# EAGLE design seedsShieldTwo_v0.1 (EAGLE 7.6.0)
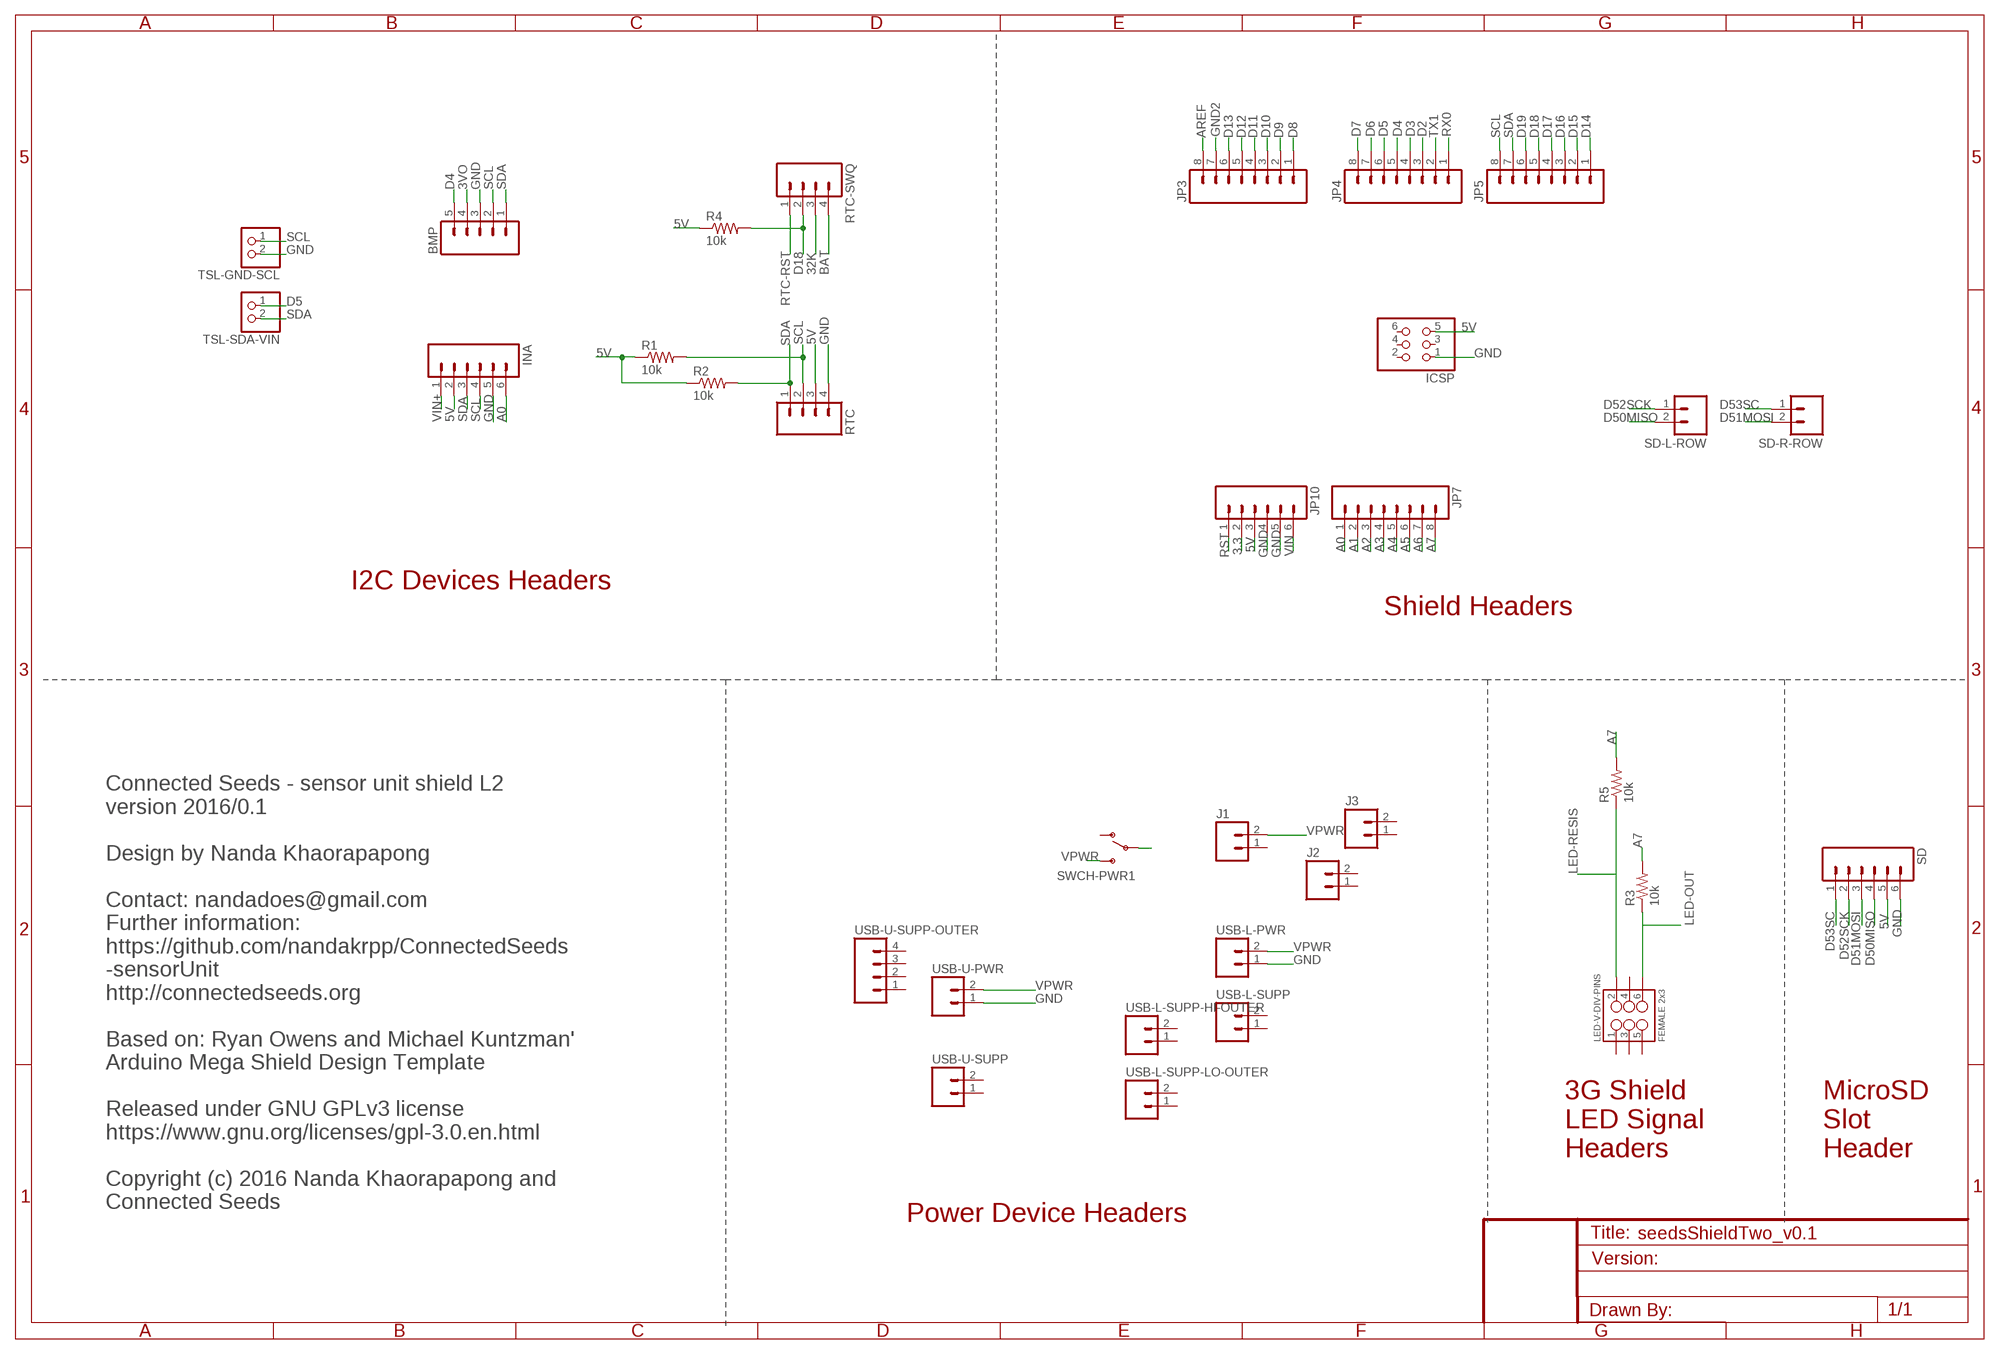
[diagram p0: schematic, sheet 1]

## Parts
BMP  M05PTH  [1X05]
ICSP  PINHD-2X3  [2X03]
INA  M06LOCK  [1X06_LOCK]
J1  M02LOCK_LONGPADS  [1X02_LOCK_LONGPADS]
J2  M02LOCK_LONGPADS  [1X02_LOCK_LONGPADS]
J3  M02LOCK_LONGPADS  [1X02_LOCK_LONGPADS]
JP3  M08LOCK  [1X08_LOCK]
JP4  M08LOCK  [1X08_LOCK]
JP5  M08LOCK  [1X08_LOCK]
JP7  M08LOCK  [1X08_LOCK]
JP10  M06LOCK  [1X06_LOCK]
LED-V-DIV-PINS  FEMALE 2x3  M03X2FEMALE  [2X3]
R1  10k  RESISTORPTH-1/4W  [AXIAL-0.4]
R2  10k  RESISTORPTH-1/4W  [AXIAL-0.4]
R3  10k  RESISTORPTH-1/4W  [AXIAL-0.4]
R4  10k  RESISTORPTH-1/4W  [AXIAL-0.4]
R5  10k  RESISTORPTH-1/4W  [AXIAL-0.4]
RTC  M04PTH  [1X04]
RTC-SWQ  M04PTH  [1X04]
SD  M06LOCK  [1X06_LOCK]
SD-L-ROW  M02PTH  [1X02]
SD-R-ROW  M02PTH  [1X02]
SWCH-PWR1  SWITCH-SPDTPTH_LOCK  [SWITCH-SPDT_LOCK.007S]
TSL-GND-SCL  JST_2PIN-THM  [JST-PH-2-THM]
TSL-SDA-VIN  JST_2PIN-THM  [JST-PH-2-THM]
USB-L-PWR  M02PTH  [1X02]
USB-L-SUPP  M02PTH  [1X02]
USB-L-SUPP-HI-OUTER  M02PTH  [1X02]
USB-L-SUPP-LO-OUTER  M02PTH  [1X02]
USB-U-PWR  M02PTH  [1X02]
USB-U-SUPP  M02PTH  [1X02]
USB-U-SUPP-OUTER  M04LOCK  [1X04_LOCK]

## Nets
3.3: JP10.2
3VO: BMP.4
5V: ICSP.5 INA.2 JP10.3 R1.P$1 R2.P$1 R4.P$1 RTC.3 SD.5
32K: RTC-SWQ.3
A0: INA.6 JP7.1
A1: JP7.2
A2: JP7.3
A3: JP7.4
A4: JP7.5
A5: JP7.6
A6: JP7.7
A7: JP7.8 R3.P$2 R5.P$2
AREF: JP3.8
BAT: RTC-SWQ.4
D2: JP4.3
D3: JP4.4
D4: BMP.5 JP4.5
D5: JP4.6 TSL-SDA-VIN.1
D6: JP4.7
D7: JP4.8
D8: JP3.1
D9: JP3.2
D10: JP3.3
D11: JP3.4
D12: JP3.5
D13: JP3.6
D14: JP5.1
D15: JP5.2
D16: JP5.3
D17: JP5.4
D18: JP5.5 R4.P$2 RTC-SWQ.2
D19: JP5.6
D50MISO: SD-L-ROW.2 SD.4
D51MOSI: SD-R-ROW.2 SD.3
D52SCK: SD-L-ROW.1 SD.2
D53SC: SD-R-ROW.1 SD.1
GND: BMP.3 ICSP.1 INA.5 JP10.4 JP10.5 RTC.4 SD.6 TSL-GND-SCL.2 USB-L-PWR.1 USB-U-PWR.1
GND2: JP3.7
LED-OUT: LED-V-DIV-PINS.6 R3.P$1
LED-RESIS: LED-V-DIV-PINS.2 R5.P$1
RST: JP10.1
RTC-RST: RTC-SWQ.1
RX0: JP4.1
SCL: BMP.2 INA.4 JP5.8 R1.P$2 RTC.2 TSL-GND-SCL.1
SDA: BMP.1 INA.3 JP5.7 R2.P$2 RTC.1 TSL-SDA-VIN.2
TX1: JP4.2
VIN: JP10.6
VIN+: INA.1 SWCH-PWR1.2(P)
VPWR: J1.2 SWCH-PWR1.3(S) USB-L-PWR.2 USB-U-PWR.2
Unconnected: ICSP.2 ICSP.3 ICSP.4 ICSP.6 J1.1 J2.1 J2.2 J3.1 J3.2 LED-V-DIV-PINS.1 LED-V-DIV-PINS.3 LED-V-DIV-PINS.4 LED-V-DIV-PINS.5 SWCH-PWR1.1(O) USB-L-SUPP-HI-OUTER.1 USB-L-SUPP-HI-OUTER.2 USB-L-SUPP-LO-OUTER.1 USB-L-SUPP-LO-OUTER.2 USB-L-SUPP.1 USB-L-SUPP.2 USB-U-SUPP-OUTER.1 USB-U-SUPP-OUTER.2 USB-U-SUPP-OUTER.3 USB-U-SUPP-OUTER.4 USB-U-SUPP.1 USB-U-SUPP.2

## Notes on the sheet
- I2C Devices Headers
- Shield Headers
- 3G Shield
  LED Signal 
  Headers
- MicroSD 
  Slot
  Header
- Connected Seeds - sensor unit shield L2 
  version 2016/0.1                                                                                                        
  
  Design by Nanda Khaorapapong                     
  
  Contact: nandadoes@gmail.com
  Further information:
  https://github.com/nandakrpp/ConnectedSeeds
  -sensorUnit
  http://connectedseeds.org
  
  Based on: Ryan Owens and Michael Kuntzman' 
  Arduino Mega Shield Design Template
  
  Released under GNU GPLv3 license
  https://www.gnu.org/licenses/gpl-3.0.en.html
  
  Copyright (c) 2016 Nanda Khaorapapong and 
  Connected Seeds
- Power Device Headers

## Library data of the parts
BMP = SparkFun-Connectors:M05: Header 5 Standard 5-pin 0.1" header. Use with straight break away headers (SKU : PRT-00116), right angle break away headers (PRT-00553), swiss pins (PRT-00743), machine pins (PRT-00117), and female headers (PRT-00115). Molex polarized connector foot print use with SKU : PRT-08230 with associated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
ICSP = SparkFun-Connectors:PINHD-2X3: PIN HEADER
INA JP10 SD = SparkFun:M06: Header 6 Standard 6-pin 0.1" header. Use with straight break away headers (SKU : PRT-00116), right angle break away headers (PRT-00553), swiss pins (PRT-00743), machine pins (PRT-00117), and female headers (PRT-00115). Molex polarized connector foot print use with SKU : PRT-08094 with associated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
J1-J3 SD-L-ROW SD-R-ROW USB-L-PWR USB-L-SUPP USB-L-SUPP-HI-OUTER USB-L-SUPP-LO-OUTER USB-U-PWR USB-U-SUPP = SparkFun-Connectors:M02: Standard 2-pin 0.1" header. Use with
JP3-JP5 JP7 = SparkFun:M08: Header 8 Standard 8-pin 0.1" header. Use with straight break away headers (SKU : PRT-00116), right angle break away headers (PRT-00553), swiss pins (PRT-00743), machine pins (PRT-00117), and female headers (PRT-00115).
LED-V-DIV-PINS = SparkFun-Connectors:M03X2: 2x3 .1" header. Shrouded, with keying- CONN-10681 SMT- CONN-11415 Pogo pins- HW-11044; PROD_ID: CONN-11566
R1-R5 = SparkFun-Passives:RESISTOR: Resistor
RTC RTC-SWQ USB-U-SUPP-OUTER = SparkFun-Connectors:M04: Header 4 Standard 4-pin 0.1" header. Use with straight break away headers (SKU : PRT-00116), right angle break away headers (PRT-00553), swiss pins (PRT-00743), machine pins (PRT-00117), and female headers (PRT-00115). Molex polarized connector foot print use with SKU : PRT-08231 with associated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; PROD_ID: CONN-09696
SWCH-PWR1 = SparkFun-Electromechanical:SWITCH-SPDT: SPDT Switch Simple slide switch, Spark Fun Electronics SKU : COM-00102 DPDT SMT slide switch, AYZ0202, SWCH-08179
TSL-GND-SCL TSL-SDA-VIN = adafruit:JST_2PIN: JST 2-Pin Connectors of various flavors

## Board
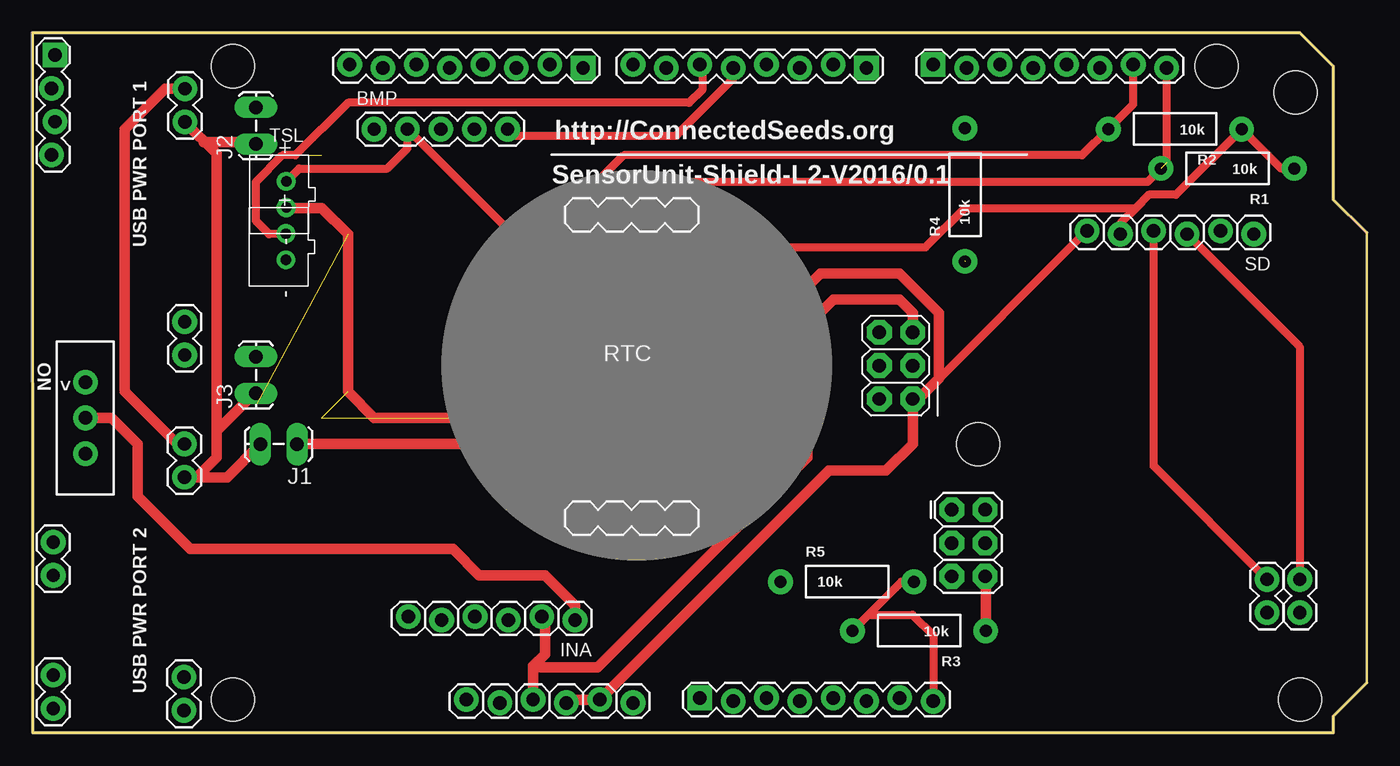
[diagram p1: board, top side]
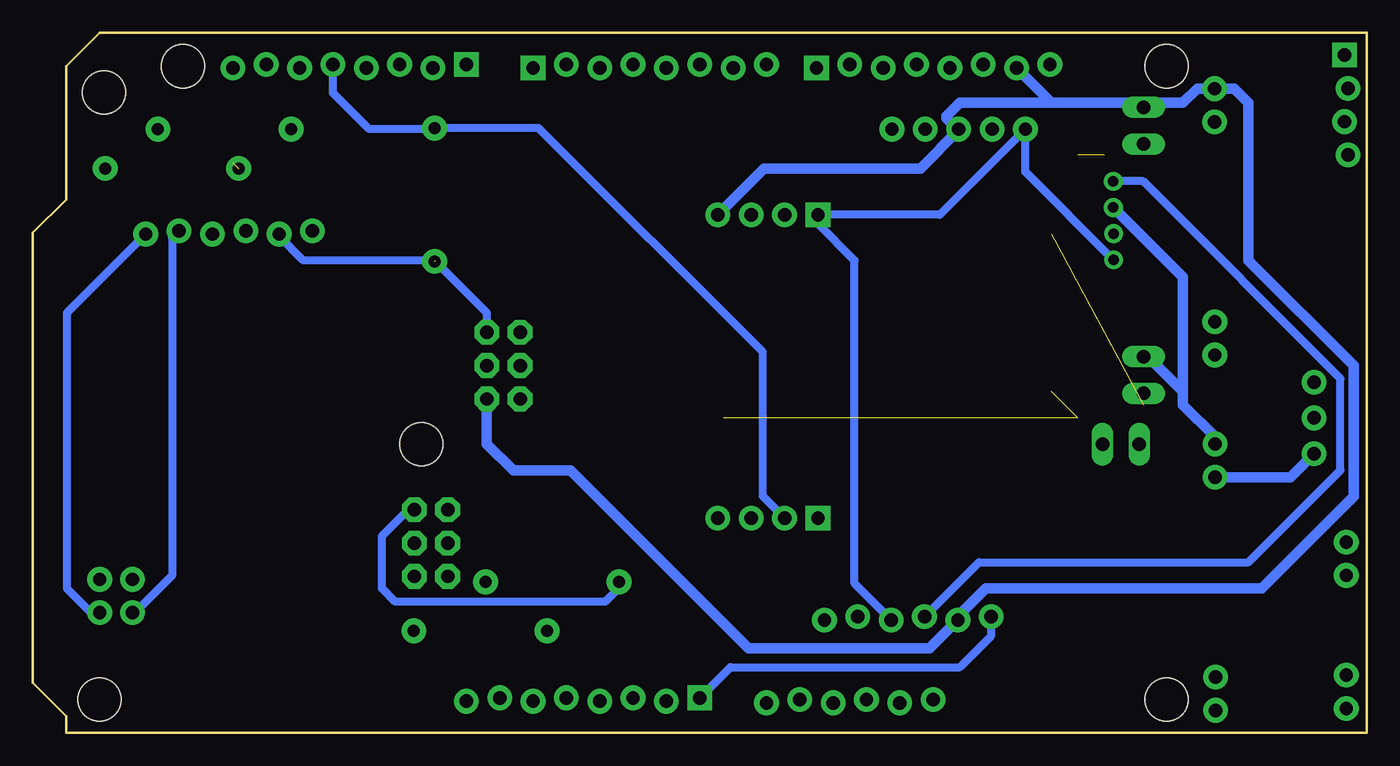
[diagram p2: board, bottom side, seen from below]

Size 101.6 x 53.34 mm. Coordinates in mm from the lower left corner, seen from the top.
Outline: 0,0 99.06,0 99.06,1.27 101.6,3.81 101.6,38.1 99.06,40.64 99.06,50.8 96.52,53.34 0,53.34 0,0
Copper layers (1*16): Top 0.035mm / dielectric 1.5mm / Bottom 0.035mm
Design rules "PCB_TRAIN": minimum track width 8mil, minimum drill 20mil, track to track 8mil, track to pad 8mil, pad to pad 8mil, via to via 8mil, smd to smd 8mil, copper to edge 10mil, drill to drill 8mil, minimum pad ring 12mil, minimum via ring 10mil, stop-mask expansion 4mil, vias tented up to drill 25mil, thermal gap 10mil

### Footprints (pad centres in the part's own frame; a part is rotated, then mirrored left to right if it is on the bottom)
1X05 = drill 1.016 pad 1.88: 1 0,0; 2 2.54,0; 3 5.08,0; 4 7.62,0; 5 10.16,0
2X03 = drill 1.016 pad 1.88 octagon: 1 -2.54,-1.27; 2 -2.54,1.27; 3 0,-1.27; 4 0,1.27; 5 2.54,-1.27; 6 2.54,1.27
1X06_LOCK = drill 1.016 pad 1.88: 1 0,0; 2 2.54,-0.254; 3 5.08,0; 4 7.62,-0.254; 5 10.16,0; 6 12.7,-0.254
1X02_LOCK_LONGPADS = drill 1.016 long: 1 -0.127,0; 2 2.667,0
1X08_LOCK = drill 1.016 pad 1.88 square: 1 0,0.127 | drill 1.016 pad 1.88: 2 2.54,-0.127; 3 5.08,0.127; 4 7.62,-0.127; 5 10.16,0.127; 6 12.7,-0.127; 7 15.24,0.127; 8 17.78,-0.127
2X3 = drill 1.016 pad 1.88 octagon: 1 0,0; 2 0,2.54; 3 2.54,0; 4 2.54,2.54; 5 5.08,0; 6 5.08,2.54
AXIAL-0.4 = drill 0.9 pad 1.88: P$1 -5.08,0; P$2 5.08,0
1X04 = drill 1.016 pad 1.88 square: 1 0,0 | drill 1.016 pad 1.88: 2 2.54,0; 3 5.08,0; 4 7.62,0
1X02 = drill 1.016 pad 1.88: 1 0,0; 2 2.54,0
SWITCH-SPDT_LOCK.007S = drill 1.016 pad 1.88: 1 0,2.718; 2 0,0; 3 0,-2.718
JST-PH-2-THM = drill 0.8 pad 1.422: 1 1,0; 2 -1,0
STAND-OFF = hole 3.302: 0,0
1X04_LOCK = drill 1.016 pad 1.88 square: 1 0,0.127 | drill 1.016 pad 1.88: 2 2.54,-0.127; 3 5.08,0.127; 4 7.62,-0.127

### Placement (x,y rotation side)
BMP  26,46 0 top
ICSP  65.75,27.98 90 top
INA  41.3,8.6 180 top
J1  20,22 180 top
J2  17,45 90 top
J3  17,26 90 top
JP3  41.91,50.8 180 top
JP4  63.5,50.8 180 top
JP5  68.58,50.8 0 top
JP7  50.8,2.54 0 top
JP10  33.02,2.54 0 top
LED-V-DIV-PINS  70,17 270 top
R1  91,43 180 top
R2  87,46 180 top
R3  67.51,7.78 180 top
R4  71,41 90 top
R5  62.03,11.51 0 top
RTC  41.8,39.48 0 top
RTC-SWQ  41.8,16.37 0 top
SD  93,38 180 top
SD-L-ROW  94,9.16 90 top
SD-R-ROW  96.5,9.16 90 top
SWCH-PWR1  4,24 0 top
TSL-GND-SCL  19.3,41.03 90 top
TSL-SDA-VIN  19.28,37.04 90 top
U$1  [STAND-OFF]  15.24,2.54 0 top
U$2  [STAND-OFF]  72,22 90 top
U$3  [STAND-OFF]  15.24,50.8 0 top
U$4  [STAND-OFF]  90.17,50.8 0 top
U$5  [STAND-OFF]  96.17,48.8 0 top
U$6  [STAND-OFF]  96.52,2.54 0 top
USB-L-PWR  11.54,22.01 270 top
USB-L-SUPP  11.52,4.26 270 top
USB-L-SUPP-HI-OUTER  1.55,4.4 270 top
USB-L-SUPP-LO-OUTER  1.55,14.54 270 top
USB-U-PWR  11.58,49.08 270 top
USB-U-SUPP  11.57,31.33 270 top
USB-U-SUPP-OUTER  1.55,51.65 270 top

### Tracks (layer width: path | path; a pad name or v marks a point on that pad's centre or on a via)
5V  (1 unrouted)
  Top 0.61: R1.P$1 95.08,43 R2.P$1 87.08,41 85,41 84,40 | 84,40 82.84,38.84 SD.5 | RTC.3 49.36,37 68,37 71,40 84,40
  Top 0.813: INA.2 39,8.61 39,6 38.1,5.1 38.1,5 | 38.1,5 JP10.3 | 38.1,5 43,5 59,21 59,31 | 21,22 50,22 59,31 | 59,31 61,33 66,33 67.02,31.98 ICSP.5
  Bottom 0.61: SD.5 82.84,37.84 81,36 71,36 67.02,32.02 ICSP.5
A0
  Bottom 0.61: JP7.1 48.47,5 31,5 28.6,7.4 INA.6
A7
  Top 0.61: R5.P$2 66.16,11.51 R3.P$2 63.65,9 67,9 68.58,7.42 JP7.8
D4
  Top 0.61: BMP.5 36.66,45.5 49,45.5 53.34,49.84 JP4.5
D5  (1 unrouted)
  Top 0.61: TSL-SDA-VIN.1 19.25,38 18,38 17,39 17,42 19,44 20,44 24,48 50,48 51,49 51,50.73 JP4.6
D18
  Bottom 0.61: R4.P$2 71.08,46 76,46 78.74,48.74 JP5.5 | 70.08,46.08 R4.P$2 | RTC-SWQ.2 46,18.03 46,29 63.08,46.08 R4.P$2
D50MISO
  Top 0.61: SD-L-ROW.2 85.38,20.32 SD.4
D51MOSI
  Top 0.61: SD.3 96.5,29.42 SD-R-ROW.2
D52SCK
  Bottom 0.61: SD.2 91,37.71 91,12 93.84,9.16 SD-L-ROW.1
D53SC
  Bottom 0.61: SD.1 99,32 99,11 97.16,9.16 SD-R-ROW.1
GND
  Top 0.61: 10.99,22.01 USB-L-PWR.1 | SD.6 67.49,25.44 ICSP.1
  Top 0.813: JP10.4 40.89,2.54 JP10.5 60.64,20 65,20 67.02,22.02 ICSP.1 | 10.99,22.01 7,26 7,46 10.08,49.08 USB-U-PWR.1
  Bottom 0.61: 31.14,8.86 INA.5
  Bottom 0.813: RTC.4 45.9,43 34,43 31.08,45.92 | 31.08,45.92 BMP.3 | 11.92,49.08 USB-U-PWR.1 | 31.08,45.92 32,46.84 32,47 31,48 24,48 | 24,48 14,48 12.92,49.08 USB-U-PWR.1 | INA.5 33.31,6.43 47.07,6.43 60.64,20 65,20 67.02,22.02 ICSP.1 | 31.14,8.86 29,11 8,11 1,18 1,28 9,36 9,48 10.08,49.08 USB-U-PWR.1 | 26.5,50.5 24,48 | TSL-GND-SCL.2 14,34.73 14,26 | USB-L-PWR.1 11.54,22.54 14,25 14,26 | 17,29 14,26
LED-OUT
  Top 0.813: LED-V-DIV-PINS.6 72.59,11.87 R3.P$1
LED-RESIS
  Bottom 0.61: LED-V-DIV-PINS.2 73,17 75,15 75,11 74,10 58,10 56.95,11.05 R5.P$1
N$6  (3 unrouted)
  Top 0.813: 67,25 69,27 69,32 66,35 60,35 49,24 26,24 24,26 24,38 22,40 20,40
N$7
  Top 0.813: 17,45 13,45
SCL  (1 unrouted)
  Top 0.61: JP5.8 86.36,43.44 84.92,42 46.86,42 RTC.2 44.34,39.34 42,37 37.54,37 BMP.2 28.54,44.54 27,43 20.27,43 TSL-GND-SCL.1
  Bottom 0.61: INA.4 29.53,13 9,13 2,20 2,27 17.03,42.03 TSL-GND-SCL.1
SDA
  Top 0.61: 84,50.75 JP5.7 83.82,47.9 R2.P$2 79.92,44 45,44 41.8,40.8 RTC.1
  Bottom 0.61: INA.3 39,11.38 39,36 41.8,38.8 RTC.1 32.52,39.48 BMP.1 26,42.75 TSL-SDA-VIN.2
VIN+
  Top 0.813: SWCH-PWR1.2 6,24 8,22 8,18 12,14 32,14 34,12 39,12 41.3,9.7 INA.1
VPWR
  Top 0.813: USB-U-PWR.2 14,44.12 14,23 | J1.2 14.8,19.47 USB-L-PWR.2 12.47,19.47 14,21 14,23 | 17,26 14,23
  Bottom 0.813: SWCH-PWR1.3 5.81,19.47 USB-L-PWR.2

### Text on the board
tPlace: TSL | http://ConnectedSeeds.org | SensorUnit-Shield-L2-V2016/0.1 | USB PWR PORT 1 | NO | < | USB PWR PORT 2
tValues: GND | 5 | 4 | 18 | 20 | 21 | VOUT | GND | SDA | SCL | GND | VIN | SDA | SCL | VCC | GND | GND | VCC | MISO | MOSI | SCK | CS | SCL | GND | VCC | GND | SDA | VOUT | RST | SQW | 32K | BAT | 50 | 51 | VCC | GND | SCL | SDA | VIN- | VIN+ | 52 | 53 | A0 | A7 | 5V | GND | GND

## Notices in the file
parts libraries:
SparkFun-Connectors: Licensing: Creative Commons ShareAlike 4.0 International - https://creativecommons.org/licenses/by-sa/4.0
